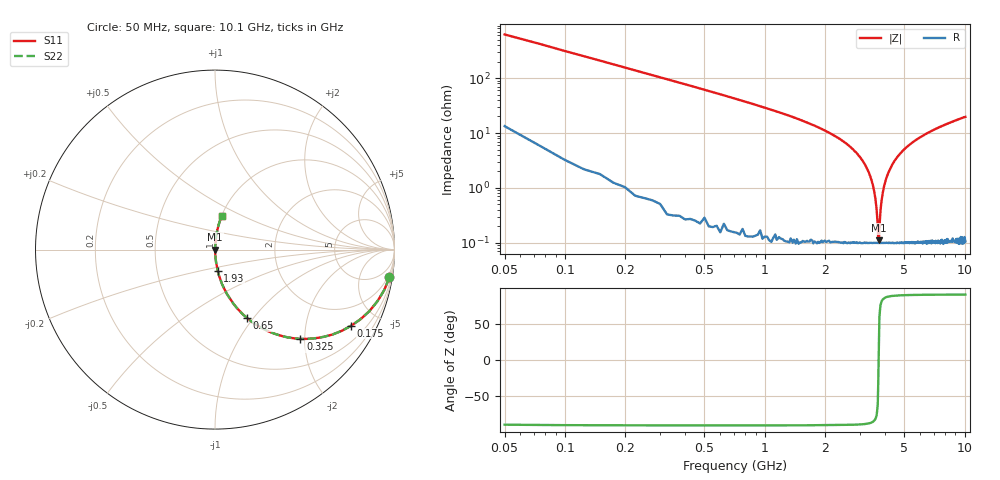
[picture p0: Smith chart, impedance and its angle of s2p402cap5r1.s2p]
! AVX Thin Film Operation		Date: April 2003
! Description: Accu-P® Series, Thin Film, SMD, RF Capacitor
! Part Number: 04025J5R1ABS
! 50 MHz  -  10.05 GHz
! Serial Measurements
# hz S db R 50
!	S11		S21		S12		S22
!	dB	Phase	dB	Phase	dB	Phase	dB	Phase
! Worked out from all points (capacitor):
!   400 points, 50 MHz to 10.1 GHz, reference 50 ohm
!   read as one part in series: C = 5.1 pF near 100 MHz
!   lowest |Z| = 111 mohm at 3.73 GHz (marker M1)
!   series resonance near 3.717 GHz, so ESL is about 360 pH
!   S11 on the Smith chart (normalised r, x): 50 MHz: 1, -12; 175 MHz: 1.03, -3.56; 325 MHz: 1.01, -1.91; 650 MHz: 1.00, -0.93; 1.93 GHz: 1.00, -0.24; 10.1 GHz: 1.00, +0.39
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5e7  -0.14 -9.1  -16.00 79.7  -16.00 79.7  -0.14 -9.1
1e8  -0.45 -17.7  -10.30 71.7  -10.30 71.7  -0.45 -17.7
1.75e8  -1.22 -29.2  -6.22 60.4  -6.22 60.4  -1.22 -29.2
3.25e8  -3.24 -46.3  -2.82 43.5  -2.82 43.5  -3.24 -46.3
6.5e8  -7.51 -64.9  -0.86 24.9  -0.86 24.9  -7.51 -64.9
1.73e9  -17.10 -81.5  -0.10 8.1  -0.10 8.1  -17.10 -81.5
1.93e9  -18.60 -82.7  -0.07 6.8  -0.07 6.8  -18.60 -82.7
2.88e9  -27.20 -86.2  -0.02 2.5  -0.02 2.5  -27.20 -86.2
3.4e9  -36.50 -85.3  -0.01 0.9  -0.01 0.9  -36.50 -85.3
3.58e9  -43.70 -80.8  -0.01 0.4  -0.01 0.4  -43.70 -80.8
3.63e9  -47.50 -76.0  -0.01 0.2  -0.01 0.2  -47.50 -76.0
3.68e9  -53.80 -60.7  -0.01 0.1  -0.01 0.1  -53.80 -60.7
3.7e9  -58.50 -33.0  -0.01 0.0  -0.01 0.0  -58.50 -33.0
3.73e9  -59.10 25.6  -0.01 -0.0  -0.01 -0.0  -59.10 25.6
3.8e9  -48.10 75.1  -0.01 -0.2  -0.01 -0.2  -48.10 75.1
3.85e9  -44.30 80.2  -0.01 -0.3  -0.01 -0.3  -44.30 80.2
4.05e9  -36.70 85.2  -0.01 -0.8  -0.01 -0.8  -36.70 85.2
4.45e9  -30.30 86.4  -0.01 -1.8  -0.01 -1.8  -30.30 86.4
5.08e9  -25.50 85.9  -0.02 -3.0  -0.02 -3.0  -25.50 85.9
6.75e9  -19.50 83.4  -0.06 -6.1  -0.06 -6.1  -19.50 83.4
8.43e9  -16.40 80.9  -0.11 -8.7  -0.11 -8.7  -16.40 80.9
1.01e10  -14.30 78.6  -0.17 -11.1  -0.17 -11.1  -14.30 78.6
